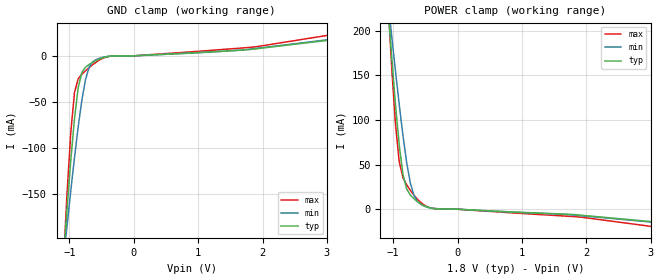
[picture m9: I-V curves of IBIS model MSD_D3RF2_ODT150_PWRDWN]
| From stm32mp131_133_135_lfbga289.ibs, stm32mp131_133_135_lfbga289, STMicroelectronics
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[Model] MSD_D3RF2_ODT150_PWRDWN
Model_type   Input
C_comp 2.506pF   2.436pF   2.576pF
Vinh = 1.150V
Vinl = 650.000mV
[Model Spec]
Vinh   1.150V   1.100V   1.200V
Vinl   650.000mV   600.000mV   700.000mV
[Temperature Range]   25.000   125.000   -40.000
[Voltage Range]   1.800V   1.700V   1.900V
[GND Clamp Reference]   0.00V   0.00V   0.00V
[POWER Clamp Reference]   1.800V   1.700V   1.900V
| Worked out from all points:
|   GND clamp passes 1 mA (typ) near -0.42 V on its own axis
|   POWER clamp passes 1 mA (typ) near -0.40 V on its own axis
[GND Clamp]
-1.785V   -950.9mA   -708.4mA   -1.315A
-1.094V   -222.1mA   -223mA     -227mA
-1.036V   -166.1mA   -184.4mA   -148.9mA
-978.8mV  -113.8mA   -146.8mA   -83.33mA
-921.2mV  -68.29mA   -110.8mA   -40.07mA
-863.6mV  -34.75mA   -77.32mA   -24.91mA
-806.1mV  -17.9mA    -47.97mA   -20mA
-748.5mV  -12.2mA    -25.39mA   -16.22mA
-690.9mV  -9.269mA   -11.95mA   -12.69mA
-575.8mV  -4.789mA   -3.741mA   -6.474mA
1.9V      7.65mA     8.034mA    9.858mA
3.57V     21.46mA    22.24mA    28.5mA
[Power Clamp]
-1.77V    962.3mA    725.2mA    1.318A
-1.079V   226mA      232.6mA    231.3mA
-1.021V   169.3mA    193.2mA    157.2mA
-963.6mV  117mA      154.8mA    95.1mA
-906.1mV  72.21mA    117.6mA    53.36mA
-848.5mV  39.42mA    82.99mA    35.44mA
-790.9mV  22.71mA    52.65mA    27.43mA
-733.3mV  15.92mA    29.39mA    21.13mA
-675.8mV  11.65mA    15.21mA    15.61mA
-560.6mV  5.32mA     5.058mA    6.918mA
-387.9mV  838.6uA    1.08mA     945uA
3.585V    -17.76mA   -18.18mA   -24.79mA
